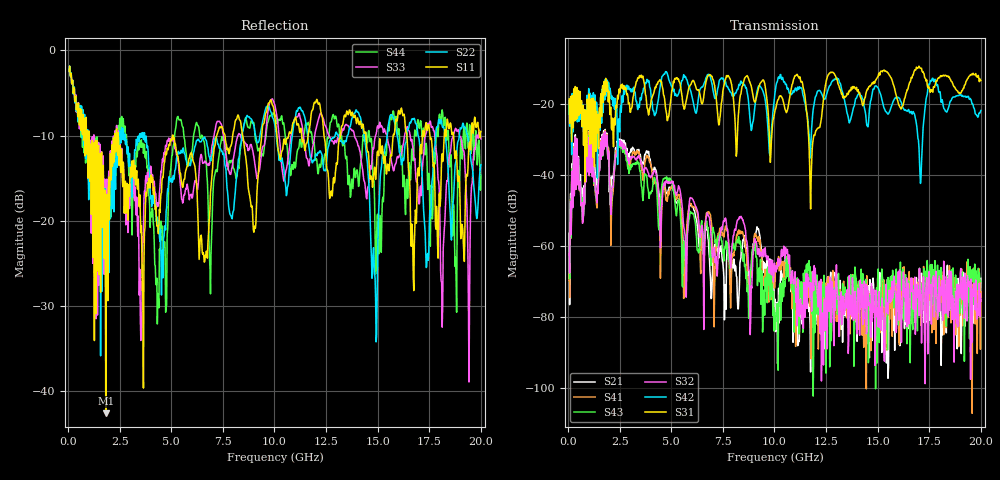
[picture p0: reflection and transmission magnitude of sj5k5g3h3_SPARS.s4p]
! FILE: E:\users\goganessyan\GBX_Backplane\FR408_backplane\1m_OUTBOUND_FEXT\sj5k5g3h3_SPARS.s4p
# MHZ S RI R 50.00
! FREQ  S11  S12  S13  S14
!  S21  S22  S23  S24
!  S31  S32  S33  S34
!  S41  S42  S43  S44
!  REAL  IMAG  REAL  IMAG  REAL  IMAG  REAL  IMAG
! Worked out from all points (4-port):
!   799 points, 50 MHz to 20 GHz, reference 50 ohm
!   strongest paths, dB at 50 MHz, 5.025 GHz, 10.03 GHz, 15.03 GHz, 20 GHz:
!     S31: -18.7, -16.3, -21.9, -12.3, -13.5
!     S42: -19.2, -15.2, -16.9, -15.6, -21.9
!     S32: -62.0, -41.7, -66.6, -82.7, -75.5
!     S43: -63.1, -42.2, -81.6, -66.4, -69.9
!     S41: -64.8, -43.7, -70.0, -82.1, -72.8
!     S21: -56.4, -43.1, -74.9, -71.5, -69.0
!   lowest |S11| = -42.6 dB at 1.825 GHz (marker M1), VSWR 1.01, Z = 50.7 + j0.341 ohm
!   |S11| at or under -10 dB: 2.433 GHz to 5.065 GHz (2.632 GHz wide, 70.2 % of centre); 5.078 GHz to 7.202 GHz (2.123 GHz wide, 34.6 % of centre); 14.43 GHz to 15.75 GHz (1.318 GHz wide, 8.73 % of centre)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
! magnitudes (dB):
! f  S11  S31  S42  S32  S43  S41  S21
! 50 MHz  -2.5  -18.7  -19.2  -62.0  -63.1  -64.8  -56.4
! 350 MHz  -5.5  -15.1  -15.4  -29.3  -29.8  -29.4  -28.7
! 1.825 GHz  -42.6  -12.8  -13.7  -31.1  -31.4  -30.7  -30.9
! 5.625 GHz  -15.1  -21.5  -12.1  -55.2  -58.7  -69.2  -60.7
! 10.05 GHz  -8.5  -21.5  -16.0  -66.3  -83.5  -65.5  -84.0
! 11.75 GHz  -8.1  -49.6  -34.2  -70.3  -69.3  -67.1  -95.4
! 20 GHz  -9.5  -13.5  -21.9  -75.5  -69.9  -72.8  -69.0
